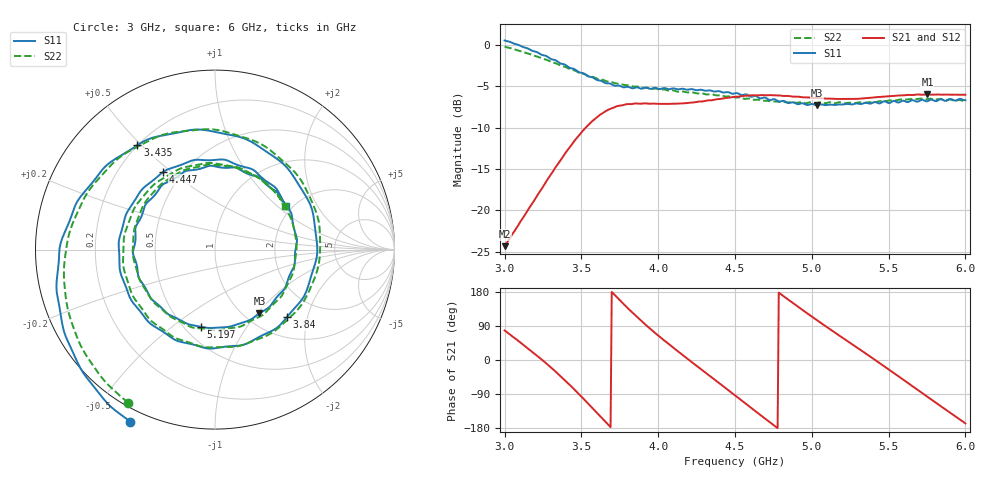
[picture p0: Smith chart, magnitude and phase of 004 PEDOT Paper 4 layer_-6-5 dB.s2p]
!  04/11/2025  19:00:46
! Ref Plane: 0.000 mm
# MHZ S MA R  50
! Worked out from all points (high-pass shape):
!   401 points, 3 GHz to 6 GHz, reference 50 ohm
!   highest |S21| = -5.96 dB at 5.753 GHz (marker M1); lowest = -24.3 dB at 3 GHz (marker M2)
!   |S21| within 3 dB of the highest: 3.586 GHz to end of sweep
!   lowest |S11| = -7.3 dB at 5.032 GHz (marker M3), VSWR 2.53, Z = 58.7 - j51.3 ohm
!   |S11| at or under -10 dB: nowhere
!   |S22| runs from -7.0 to -0.2 dB; largest |S21 - S12| = 0.012
!   S11 on the Smith chart (normalised r, x): 3 GHz: -0.05, -0.62; 3.435 GHz: 0.20, +0.49; 3.84 GHz: 1.40, -1.50; 4.447 GHz: 0.39, +0.47; 5.197 GHz: 0.60, -0.64; 6 GHz: 1.85, +1.15
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3000  1.068 -116.2  0.06069 77.8  0.06114 78.9  0.9813 -119.6
3217.5  0.9011 -168.4  0.1251 9.4  0.1253 10.4  0.8505 -171.8
3330  0.8124 160.6  0.1814 -29.9  0.1816 -29.1  0.7794 156.5
3435  0.7248 126.6  0.2485 -70.0  0.2492 -69.5  0.7103 122.2
3502.5  0.6803 101.9  0.2981 -97.5  0.2983 -96.9  0.6739 97.1
3585  0.6283 68.8  0.3558 -132.4  0.3577 -131.8  0.6385 63.8
3682.5  0.5869 25.1  0.4099 -173.9  0.4105 -173.2  0.6009 21.3
3840  0.5495 -43.1  0.4422 122.0  0.4423 123.0  0.5616 -44.6
4005  0.5431 -101.7  0.4413 63.1  0.4412 64.0  0.539 -103.2
4222.5  0.5418 -168.2  0.4494 -6.8  0.4509 -6.0  0.5186 -170.5
4447.5  0.5202 123.6  0.4801 -77.0  0.4821 -76.0  0.4889 119.7
4500  0.5113 106.8  0.4872 -93.4  0.4894 -92.5  0.4826 103.1
4627.5  0.4931 66.0  0.4973 -133.3  0.4972 -132.7  0.467 61.2
4747.5  0.4705 27.7  0.497 -170.8  0.4968 -169.9  0.4571 21.9
4867.5  0.4504 -8.8  0.4899 153.1  0.489 154.1  0.4532 -16.0
5002.5  0.4402 -46.9  0.4797 114.0  0.4788 114.8  0.4497 -55.8
5032.5  0.433 -55.1  0.4785 105.4  0.4782 106.2  0.4454 -65.1
5197.5  0.4374 -100.4  0.472 59.5  0.4715 60.2  0.4487 -110.3
5362.5  0.4461 -145.8  0.4786 14.1  0.4787 14.8  0.4502 -154.5
5505  0.4463 172.8  0.4912 -26.0  0.4925 -24.9  0.4628 167.4
5752.5  0.4577 100.3  0.5037 -97.0  0.5055 -95.8  0.4717 98.8
6000  0.4643 31.6  0.5008 -167.3  0.5017 -166.5  0.4567 31.8
